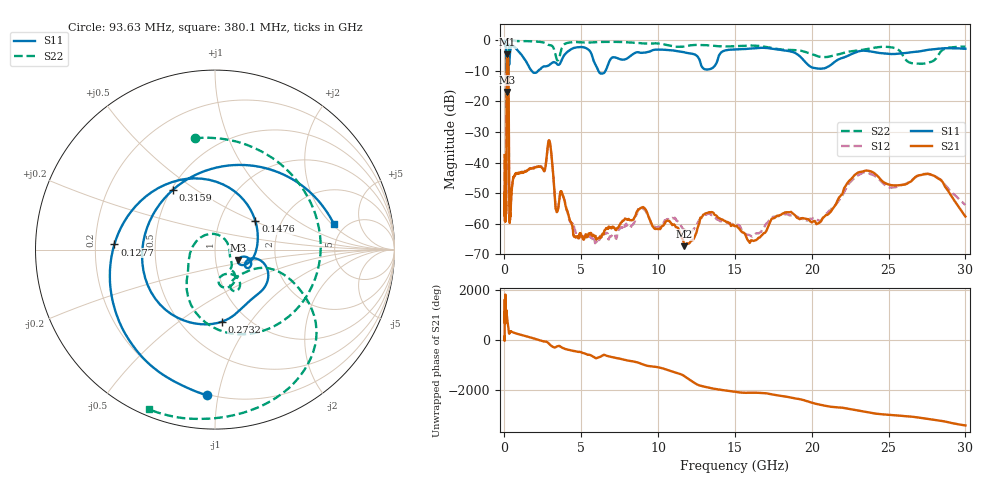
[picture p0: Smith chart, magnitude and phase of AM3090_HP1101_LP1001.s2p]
! Date/Time: Thu, Feb 28, 2019 2:08 PM
! Network Analyzer: Agilent Technologies E8364B Rev: A.07.50.67
! Sweep from 0.010 to 30.000 GHz, 1601 Points, Sweep Type: LOG
! Power Supply: 5.022 V, 0.002 A
# Hz S DB R 50
!freq MagS11 AngS11 MagS21 AngS21 MagS12 AngS12 MagS22 AngS22
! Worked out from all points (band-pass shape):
!   1601 points, 10 MHz to 30 GHz, reference 50 ohm
!   highest |S21| = -4.65 dB at 197.3 MHz (marker M1); lowest = -67.3 dB at 11.71 GHz (marker M2)
!   |S21| within 3 dB of the highest: 152 MHz to 254.5 MHz (102.5 MHz wide, 50.4 % of centre)
!   lowest |S11| = -17.0 dB at 173.3 MHz (marker M3), VSWR 1.33, Z = 64.3 - j7.55 ohm
!   |S11| at or under -10 dB: 144.3 MHz to 232.4 MHz (88.15 MHz wide, 46.8 % of centre); 1.763 GHz to 2.202 GHz (439.2 MHz wide, 22.2 % of centre); 6.111 GHz to 6.583 GHz (472.1 MHz wide, 7.44 % of centre)
!   |S22| runs from -22.1 to -0.1 dB; largest |S21 - S12| = 0.016
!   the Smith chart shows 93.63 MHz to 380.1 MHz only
!   S11 on the Smith chart (normalised r, x): 93.63 MHz: 0.19, -0.93; 127.7 MHz: 0.28, +0.02; 147.6 MHz: 1.48, +0.50; 273.2 MHz: 0.77, -0.74; 315.9 MHz: 0.51, +0.41; 380.1 MHz: 4.02, +2.12
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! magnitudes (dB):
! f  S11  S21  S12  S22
! 10 MHz  -0.3  -37.6  -39.2  -0.6
! 38.04 MHz  -0.4  -58.0  -57.1  -1.4
! 93.63 MHz  -1.8  -55.4  -54.9  -4.0
! 115.5 MHz  -3.3  -52.9  -53.8  -4.6
! 127.7 MHz  -5.0  -38.4  -38.0  -5.2
! 144.7 MHz  -10.2  -11.8  -11.8  -19.6
! 147.6 MHz  -11.2  -9.6  -9.6  -21.5
! 173.3 MHz  -17.0  -5.0  -5.0  -16.2
! 197.3 MHz  -13.3  -4.6  -4.6  -13.3
! 273.2 MHz  -7.9  -16.1  -16.0  -7.9
! 315.9 MHz  -7.8  -54.7  -55.9  -0.8
! 380.1 MHz  -3.4  -57.3  -56.0  -0.3
! 550.5 MHz  -2.0  -45.7  -45.8  -0.2
! 2.084 GHz  -10.6  -41.5  -41.4  -0.5
! 2.928 GHz  -8.1  -32.9  -32.9  -1.6
! 3.385 GHz  -7.6  -56.0  -56.1  -6.0
! 4.663 GHz  -2.4  -64.5  -63.5  -0.6
! 7.926 GHz  -6.2  -58.5  -60.0  -0.7
! 11.71 GHz  -4.0  -67.3  -61.9  -2.1
! 20.41 GHz  -9.3  -59.9  -58.9  -5.3
! 23.36 GHz  -3.5  -42.9  -43.2  -3.2
! 30 GHz  -2.8  -57.6  -53.9  -2.2
